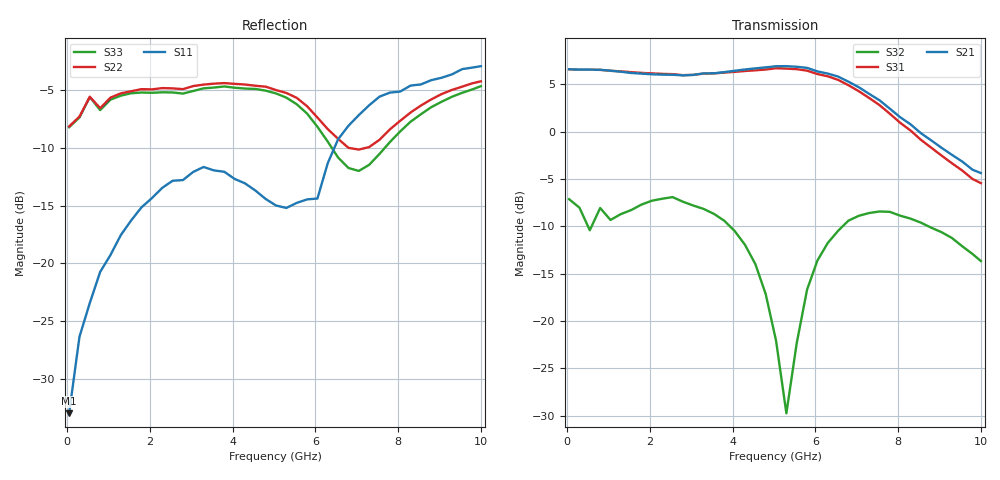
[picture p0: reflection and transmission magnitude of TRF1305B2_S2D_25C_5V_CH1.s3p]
! Created Wed Jul  2 22:02:46 2025
# hz S ma R 50
! 3 Port Network Data from SP1.SP block
! PORT[1] = INP
! PORT[2]= OUTM
! PORT[3] = OUTP
! freq  magS11  angS11  magS12  angS12  magS13  angS13
!  magS21  angS21
!  magS22  angS22  magS23  angS23
!  magS31  angS31  magS32  angS32
!  magS33  angS33
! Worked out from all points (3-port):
!   41 points, 50 MHz to 10 GHz, reference 50 ohm
!   strongest paths, dB at 50 MHz, 2.55 GHz, 5.05 GHz, 7.55 GHz, 10 GHz:
!     S21: 6.6, 6.0, 6.9, 3.3, -4.4
!     S31: 6.6, 6.1, 6.7, 2.8, -5.4
!     S32: -7.1, -6.9, -22.1, -8.4, -13.7
!   lowest |S11| = -33.0 dB at 50 MHz (marker M1), VSWR 1.05, Z = 47.9 - j0.505 ohm
!   |S11| at or under -10 dB: start of sweep to 6.46 GHz
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5e7  0.02242 -166.4  0.003354 21.0  0.001726 118.3
     2.13 177.8  0.3917 175.5  0.4378 1.5
     2.131 -2.1  0.4394 1.8  0.3885 174.8
5.5e8  0.06736 -124.1  0.02164 61.9  0.01729 68.2
       2.121 159.2  0.5264 162.3  0.3031 -6.7
       2.118 -20.2  0.3013 -6.8  0.5252 162.8
2.55e9  0.2278 -140.8  0.04023 7.9  0.02279 -31.7
        1.993 88.3  0.5725 81.8  0.4537 -24.3
        2.008 -90.8  0.4508 -23.6  0.5496 83.2
4.05e9  0.232 -164.4  0.06328 -5.5  0.02205 -75.2
        2.092 36.7  0.5988 44.6  0.3069 -66.8
        2.064 -143.3  0.2988 -64.4  0.5762 44.5
5.05e9  0.178 -164.9  0.09683 -35.9  0.03082 -115.5
        2.211 -4.3  0.5628 23.4  0.07951 -133.4
        2.157 175.6  0.07891 -116.2  0.5442 20.1
5.3e9  0.1737 -162.8  0.1036 -45.4  0.03173 -128.8
       2.212 -15.9  0.5468 18.4  0.05494 151.4
       2.148 164.1  0.0326 166.6  0.5219 14.3
6.55e9  0.3447 -146.2  0.113 -85.4  0.02309 154.2
        1.949 -74.5  0.3461 6.7  0.3256 34.3
        1.873 104.0  0.2994 33.4  0.2872 1.0
7.8e9  0.5488 -175.3  0.1049 -124.6  0.01109 90.0
       1.32 -128.7  0.3801 29.0  0.3816 -7.5
       1.241 48.0  0.3768 -8.0  0.335 30.8
9.3e9  0.6581 159.6  0.0849 -156.4  0.002502 125.0
       0.7534 -175.3  0.5636 15.7  0.285 -36.0
       0.6803 -1.3  0.2744 -37.6  0.5263 16.6
1e10  0.7143 151.9  0.07885 -170.2  0.004967 110.9
      0.6037 166.8  0.6142 5.2  0.2211 -45.6
      0.5341 -20.4  0.2074 -46.9  0.5851 6.3
